{attribute 'qualified_only'}
{attribute 'strict'}
FUNCTION_BLOCK FB_WithMethods
VAR_INPUT
    bExecute : BOOL;
END_VAR
VAR_OUTPUT
    bBusy : BOOL;
    bError : BOOL;
    nErrorId : UDINT;
END_VAR
VAR
    _counter : INT;
    _initialized : BOOL;
END_VAR

(* Main implementation *)
IF bExecute AND NOT _initialized THEN
    Initialize();
END_IF

METHOD PUBLIC Initialize : BOOL
VAR_INPUT
    nStartValue : INT := 0;
END_VAR
VAR
    i : INT;
END_VAR
FOR i := 0 TO 10 DO
    _counter := _counter + 1;
END_FOR
_initialized := TRUE;
Initialize := TRUE;
END_METHOD

METHOD PRIVATE Reset
VAR
    temp : INT;
END_VAR
_counter := 0;
_initialized := FALSE;
END_METHOD

METHOD Calculate : REAL
VAR_INPUT
    fInput : REAL;
END_VAR
VAR_OUTPUT
    fOutput : REAL;
END_VAR
VAR
    fTemp : REAL;
END_VAR
CASE _counter OF
    0:
        fTemp := 0.0;
    1..5:
        fTemp := fInput * 2.0;
    6, 7, 8:
        fTemp := fInput / 2.0;
ELSE
    fTemp := fInput;
END_CASE

fOutput := fTemp;
Calculate := fTemp;
END_METHOD

END_FUNCTION_BLOCK
